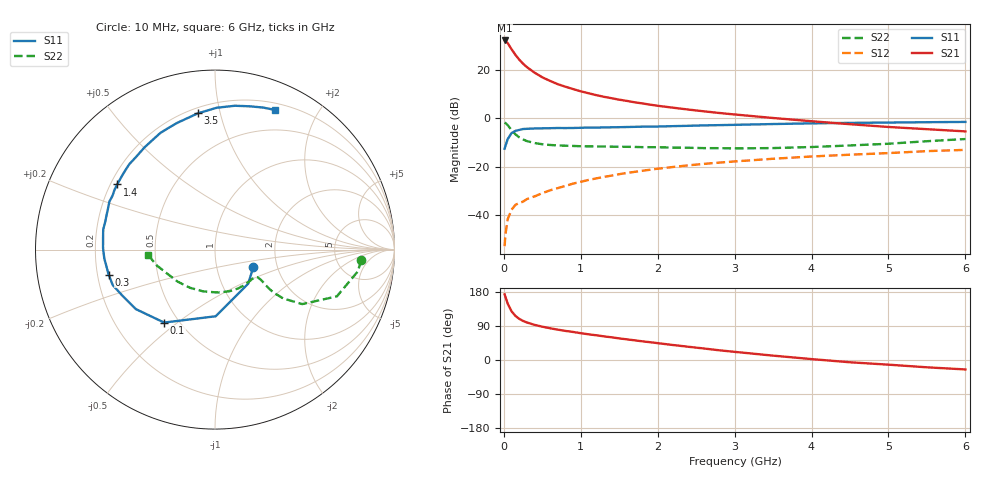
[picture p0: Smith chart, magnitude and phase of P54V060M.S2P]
! SIEMENS Small Signal Semiconductors
! BFP183
! Si NPN RF Bipolar Junction Transistor in SOT143
! VCE = 4 V  IC = 60 mA
! Common Emitter S-Parameters:  March  1996
# GHz  S  MA  R  50
!  f  S11  S21  S12  S22
! GHz  MAG  ANG  MAG  ANG  MAG  ANG  MAG  ANG
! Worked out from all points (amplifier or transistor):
!   36 points, 10 MHz to 6 GHz, reference 50 ohm
!   highest |S21| = 32.5 dB at 10 MHz (marker M1)
!   |S21| within 3 dB of that: start of sweep to 87.4 MHz
!   unconditionally stable (mu >= 1): start of sweep to 21.38 MHz; 259.5 MHz to end of sweep
!   at 250 MHz: K = 0.99, MSG = 28.7 dB, |S12| = -34.6 dB
!   at 1.4 GHz: K = 1.49, MAG = 12.0 dB, |S12| = -23.8 dB
!   at 6 GHz: K = 1.14, MAG = 1.6 dB, |S12| = -13.1 dB
!   S11 on the Smith chart (normalised r, x): 10 MHz: 1.50, -0.31; 100 MHz: 0.42, -0.45; 300 MHz: 0.25, -0.11; 1.4 GHz: 0.23, +0.29; 3.5 GHz: 0.23, +0.85; 6 GHz: 0.27, +1.49
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0.01  0.235 -24.8  41.98 173.2  0.0022 68.0  0.8179 -4.1
0.02  0.265 -45.7  41.4 166.8  0.0038 73.1  0.804 -8.8
0.05  0.3715 -89.4  36.96 148.9  0.008 66.9  0.7272 -21.0
0.1  0.4956 -124.9  27.62 128.7  0.0126 52.4  0.5731 -32.0
0.15  0.5514 -143.0  21.15 116.4  0.0159 50.0  0.4682 -35.6
0.2  0.5768 -153.7  16.79 108.7  0.0174 49.9  0.4051 -36.3
0.25  0.6031 -160.9  13.78 103.0  0.0186 50.2  0.3654 -35.7
0.3  0.6087 -166.8  11.71 99.1  0.021 51.3  0.3382 -34.7
0.4  0.6187 -175.4  8.954 92.6  0.0239 55.9  0.3078 -33.4
0.5  0.6238 179.2  7.183 87.9  0.0279 56.7  0.291 -33.1
0.6  0.627 174.1  6.058 83.8  0.0319 58.8  0.2808 -33.2
0.7  0.6328 169.8  5.176 80.1  0.0355 59.9  0.2745 -33.7
0.8  0.6309 165.8  4.575 76.8  0.0394 61.1  0.2708 -34.9
1.1  0.6464 155.5  3.349 67.8  0.0525 61.3  0.2628 -39.4
1.4  0.6548 146.3  2.638 59.9  0.0646 60.5  0.2587 -45.3
1.7  0.669 137.5  2.171 51.9  0.0774 58.5  0.2555 -52.3
2.2  0.6918 124.6  1.674 39.5  0.0977 54.2  0.2474 -65.0
2.8  0.7263 110.7  1.301 25.6  0.1205 48.4  0.2409 -82.8
3.5  0.7651 97.2  1.022 11.5  0.145 41.7  0.242 -106.1
4.5  0.8091 82.1  0.759 -6.0  0.1762 31.7  0.2743 -139.5
5.5  0.8355 71.3  0.598 -19.3  0.209 22.7  0.3363 -164.8
6  0.8471 66.7  0.538 -24.9  0.222 17.7  0.3732 -175.3
